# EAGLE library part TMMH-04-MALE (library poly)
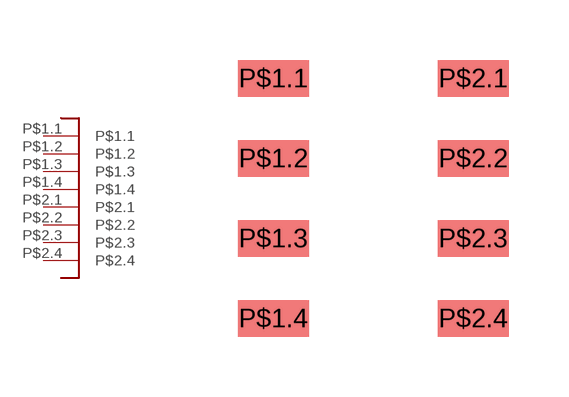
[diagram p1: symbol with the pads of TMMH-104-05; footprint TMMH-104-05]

Designator prefix -

## TMMH-04-MALE  [TMMH-104-05]
P$1.1  P$1.1
P$1.2  P$1.2
P$1.3  P$1.3
P$1.4  P$1.4
P$2.1  P$2.1
P$2.2  P$2.2
P$2.3  P$2.3
P$2.4  P$2.4

## Footprint TMMH-104-05 (pad centres in mm)
smd 1.778 x 0.914: P$1.1 -2.5,2; P$1.2 -2.5,0; P$1.3 -2.5,-2; P$1.4 -2.5,-4; P$2.1 2.5,2; P$2.2 2.5,0; P$2.3 2.5,-2; P$2.4 2.5,-4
